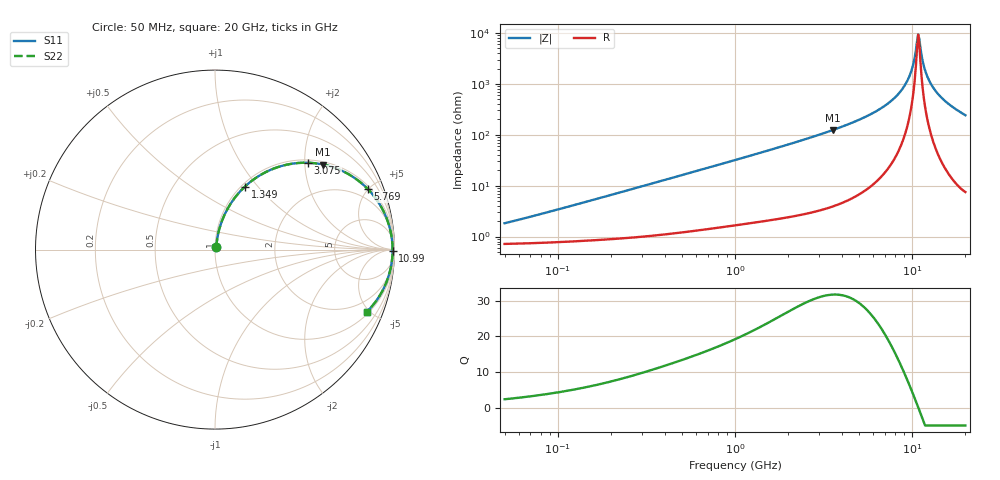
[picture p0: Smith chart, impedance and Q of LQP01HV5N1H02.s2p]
!Murata Part Number: LQP01HV5N1H02
!These Parameters are Measured in Series Mode Connection
!  o--[Z]--o
!Port1  Port2
!  o-------o
!Freq. Start=50[MHz] Stop=20[GHz], 401[Steps]
# Hz S RI R 50
!Freq.(Hz) S11(Real) S11(Imag) S21(Real) S21(Imag) S12(Real) S12(Imag) S22(Real) S22(Imag)
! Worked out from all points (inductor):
!   401 points, 50 MHz to 20 GHz, reference 50 ohm
!   read as one part in series: L = 5.31 nH near 66.46 MHz
!   highest Q = 31.7 at 3.572 GHz (marker M1), where L = 5.52 nH
!   self-resonance near 10.82 GHz
!   S11 on the Smith chart (normalised r, x): 50 MHz: 1.01, +0.03; 1.349 GHz: 1.04, +0.86; 3.075 GHz: 1.07, +2.07; 5.769 GHz: 1.19, +4.96; 10.99 GHz: open; 20 GHz: 1.15, -4.84
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5e7  0.0074 0.0166  0.9926 -0.0166  0.9926 -0.0166  0.0074 0.0166
1.364002e8  0.0101 0.0442  0.9899 -0.0442  0.9899 -0.0442  0.0101 0.0442
3.721004e8  0.0244 0.1159  0.9756 -0.1159  0.9756 -0.1159  0.0244 0.1159
1e9  0.104 0.2802  0.896 -0.2802  0.896 -0.2802  0.104 0.2802
1.349283e9  0.1668 0.351  0.8332 -0.351  0.8332 -0.351  0.1668 0.351
1.904239e9  0.2803 0.4306  0.7197 -0.4306  0.7197 -0.4306  0.2803 0.4306
2.728004e9  0.4513 0.4814  0.5487 -0.4814  0.5487 -0.4814  0.4513 0.4814
3.075291e9  0.5175 0.4839  0.4825 -0.4839  0.4825 -0.4839  0.5175 0.4839
3.572216e9  0.603 0.4737  0.397 -0.4737  0.397 -0.4737  0.603 0.4737
5.769027e9  0.8511 0.3376  0.1489 -0.3376  0.1489 -0.3376  0.8511 0.3376
7.442007e9  0.9388 0.2141  0.0612 -0.2141  0.0612 -0.2141  0.9388 0.2141
8.516016e9  0.9682 0.1401  0.0318 -0.1401  0.0318 -0.1401  0.9682 0.1401
9.316812e9  0.9809 0.0888  0.0191 -0.0888  0.0191 -0.0888  0.9809 0.0888
1.004137e10  0.9872 0.0453  0.0128 -0.0453  0.0128 -0.0453  0.9872 0.0453
1.066139e10  0.9893 0.01  0.0107 -0.01  0.0107 -0.01  0.9893 0.01
1.082228e10  0.9895 0.00121  0.0105 -0.00121  0.0105 -0.00121  0.9895 0.00121
1.098561e10  0.9895 -0.00763  0.0105 0.00763  0.0105 0.00763  0.9895 -0.00763
1.183995e10  0.987 -0.0519  0.013 0.0519  0.013 0.0519  0.987 -0.0519
1.238412e10  0.9835 -0.0784  0.0165 0.0784  0.0165 0.0784  0.9835 -0.0784
1.314879e10  0.9766 -0.1137  0.0234 0.1137  0.0234 0.1137  0.9766 -0.1137
1.573793e10  0.9395 -0.2172  0.0605 0.2172  0.0605 0.2172  0.9395 -0.2172
2e10  0.8465 -0.3453  0.1535 0.3453  0.1535 0.3453  0.8465 -0.3453
